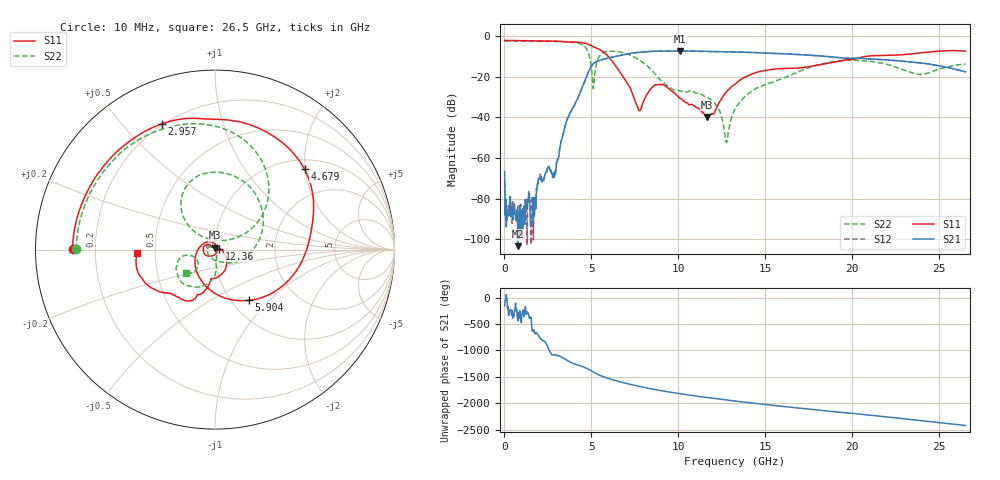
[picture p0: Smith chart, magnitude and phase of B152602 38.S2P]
!  2-Port S-parameters saved by WinCal
! VAR MeasName=S-Parameters (CALIBRATED_DATA) read from VNA (N5242A)
! VAR MeasDate=2016-1-5 16:31:39
! VAR NAME=B152602 38
! VAR FILENAME=B152602 38.S2P
! VAR DATE=2016-1-5 16:31:39
! VAR PHYS_PORTS=1,2
# Hz S DB R 50
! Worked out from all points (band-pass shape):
!   801 points, 10 MHz to 26.5 GHz, reference 50 ohm
!   highest |S21| = -7.19 dB at 10.11 GHz (marker M1); lowest = -103.5 dB at 771.6 MHz (marker M2)
!   |S21| within 3 dB of the highest: 6.211 GHz to 18.87 GHz (12.66 GHz wide, 101 % of centre)
!   lowest |S11| = -39.8 dB at 11.67 GHz (marker M3), VSWR 1.02, Z = 50 + j1.02 ohm
!   |S11| at or under -10 dB: 5.977 GHz to 20.66 GHz (14.69 GHz wide, 110 % of centre)
!   |S22| runs from -52.4 to -2.2 dB; largest |S21 - S12| = 0.0028
!   S11 on the Smith chart (normalised r, x): 10 MHz: 0.12, +0.00; 2.957 GHz: 0.19, +0.64; 4.679 GHz: 1.22, +1.98; 5.904 GHz: 1.20, -0.77; 12.36 GHz: 1.05, +0.01; 26.5 GHz: 0.40, -0.02
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1e7  -2.01 179.7  -66.63 -155.1  -71.84 -94.7  -2.23 179.9
1.755625e8  -2.02 176.4  -85.62 147.2  -89.42 -0.0  -2.24 177.3
7.715875e8  -2.08 164.1  -103.45 -78.5  -83.75 -149.3  -2.28 168.1
1.665625e9  -2.19 145.4  -86.02 77.5  -100.43 106.6  -2.35 153.9
2.029862e9  -2.23 137.2  -69.52 -34.5  -69.81 -39.5  -2.39 147.7
2.957012e9  -2.37 113.1  -65.91 3.2  -64.06 9.7  -2.51 129.7
3.553038e9  -2.74 94.3  -42.18 -97.6  -42.24 -97.4  -2.68 114.9
4.447075e9  -3.08 56.0  -25.78 139.5  -25.79 139.5  -3.90 76.5
4.678862e9  -3.47 41.9  -20.67 108.9  -20.69 109.1  -5.60 57.4
5.109325e9  -5.08 13.8  -13.54 30.9  -13.54 31.1  -25.78 81.4
5.904025e9  -9.35 -56.1  -10.80 -81.6  -10.78 -81.5  -7.40 99.7
7.725212e9  -36.46 12.1  -7.85 121.3  -7.85 121.3  -11.54 16.6
8.851038e9  -23.69 -174.3  -7.32 48.1  -7.30 48.0  -20.44 -50.1
1.010931e10  -30.56 136.3  -7.19 -20.1  -7.18 -20.1  -26.89 -149.5
1.16656e10  -39.80 87.6  -7.41 -92.3  -7.40 -92.1  -30.20 150.2
1.236096e10  -32.40 14.5  -7.50 -121.4  -7.49 -121.3  -36.64 123.4
1.275831e10  -27.41 -8.9  -7.58 -137.6  -7.60 -137.5  -52.44 37.7
1.3255e10  -23.55 -29.2  -7.68 -157.1  -7.68 -157.1  -35.75 -64.5
1.557288e10  -16.08 -86.9  -8.40 116.4  -8.38 116.3  -22.01 -85.7
1.769208e10  -14.65 -98.8  -9.37 42.0  -9.34 42.2  -14.97 -98.0
2.209604e10  -9.33 -131.8  -11.67 -102.3  -11.61 -102.7  -14.02 -166.6
2.65e10  -7.26 -177.9  -17.49 100.6  -17.51 100.4  -13.63 -142.0
